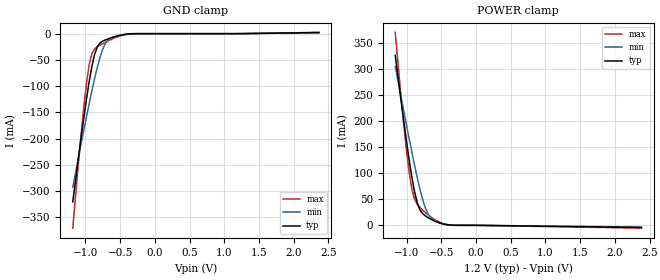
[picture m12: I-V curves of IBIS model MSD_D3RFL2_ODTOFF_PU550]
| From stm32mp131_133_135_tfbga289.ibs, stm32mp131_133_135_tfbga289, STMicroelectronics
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[Model] MSD_D3RFL2_ODTOFF_PU550
Model_type   Input
C_comp 2.435pF   2.348pF   2.561pF
Vinh = 820.000mV
Vinl = 380.000mV
[Temperature Range]   25.000   125.000   -40.000
[Voltage Range]   1.200V   1.140V   1.300V
[GND Clamp Reference]   0.00V   0.00V   0.00V
[POWER Clamp Reference]   1.200V   1.140V   1.300V
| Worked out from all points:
|   GND clamp passes 1 mA (typ) near -0.40 V on its own axis
|   POWER clamp passes 1 mA (typ) near -0.41 V on its own axis
[GND Clamp]
-1.182V   -320.2mA   -292.6mA   -370.3mA
-1.064V   -199.8mA   -211.1mA   -194.2mA
-984.9mV  -125.2mA   -158.4mA   -95.11mA
-945.5mV  -91.49mA   -133mA     -59.06mA
-906.1mV  -62.07mA   -108.5mA   -37.48mA
-866.7mV  -39.14mA   -85.09mA   -28.62mA
-787.9mV  -17.47mA   -44.46mA   -21.6mA
-709.1mV  -11.73mA   -17.93mA   -16.13mA
-630.3mV  -8.05mA    -7.634mA   -11.12mA
-512.1mV  -3.598mA   -3.037mA   -4.835mA
-275.8mV  -45.79uA   -87.99uA   -33.99uA
2.364V    2.082mA    1.757mA    2.454mA
[Power Clamp]
-1.164V   326.7mA    305.4mA    371mA
-1.085V   244.4mA    250mA      252.9mA
-1.006V   165.3mA    195.3mA    148.3mA
-966.7mV  128.4mA    168.4mA    105mA
-927.3mV  94.69mA    142.1mA    71.68mA
-887.9mV  65.78mA    116.6mA    51.25mA
-809.1mV  29.89mA    69.68mA    34.44mA
-730.3mV  18.15mA    33.48mA    24.45mA
-690.9mV  14.77mA    21.68mA    20.09mA
-572.7mV  6.926mA    6.826mA    9.285mA
-336.4mV  199.6uA    379.1uA    222.8uA
2.382V    -4.167mA   -3.304mA   -5.413mA
